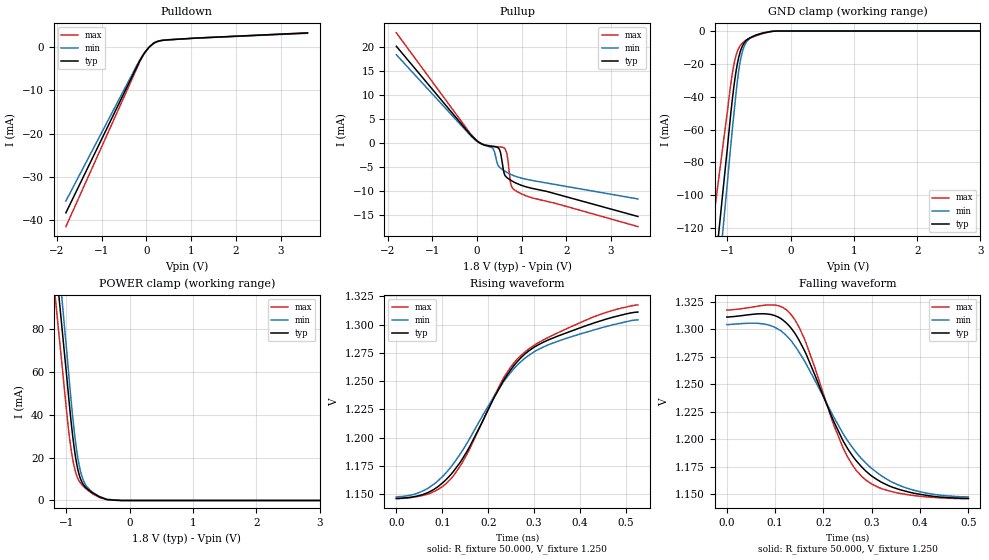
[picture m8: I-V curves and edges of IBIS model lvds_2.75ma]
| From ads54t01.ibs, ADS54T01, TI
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[Model]   lvds_2.75ma
Model_type 3-state
Vref=1.250E+00
Rref=5.000E+01
Cref=0.000E+00
Vmeas=1.250E+00
C_comp   7.860E-13   7.790E-13   7.930E-13
[Voltage Range]   1.800E+00   1.650E+00   1.950E+00
[POWER Clamp Reference]   1.800E+00   1.650E+00   1.950E+00
[GND Clamp Reference]   0.000E+00   0.000E+00   0.000E+00
[Pullup Reference]   1.800E+00   1.650E+00   1.950E+00
[Pulldown Reference]   0.000E+00   0.000E+00   0.000E+00
[Temperature Range]   25   85   -40
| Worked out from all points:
|   slope of the pulldown table from 0 to 0.27 V, typ, clamps not added: 125 ohm
|   slope of the pullup table from 0 to 0.27 V, typ, clamps not added: 263 ohm
|   GND clamp passes 1 mA (typ) near -0.41 V on its own axis
|   POWER clamp passes 1 mA (typ) near -0.41 V on its own axis
|   rising waveform, R_fixture 50.000, V_fixture 1.250: 20-80 % time 153ps typ, 161ps min, 159ps max; typ from 1.15 V to 1.31 V
|   falling waveform, R_fixture 50.000, V_fixture 1.250: 20-80 % time 107ps typ, 128ps min, 87.4ps max; typ from 1.31 V to 1.15 V
[GND Clamp]
-1.8V     -374.4mA   -423.5mA   -288.4mA
-1.02V    -78.69mA   -100.5mA   -54.92mA
-920mV    -41.17mA   -59.34mA   -25.51mA
-860mV    -23.88mA   -36.88mA   -14.48mA
-820mV    -15.94mA   -23.97mA   -10.43mA
-780mV    -10.76mA   -15.27mA   -8.038mA
-740mV    -7.589mA   -9.923mA   -6.562mA
-700mV    -5.657mA   -6.755mA   -5.499mA
-640mV    -4.069mA   -4.329mA   -4.359mA
-460mV    -1.489mA   -1.354mA   -1.806mA
-220mV    -4.201uA   -14.01uA   -11.29uA
3.6V      0A         0A         0A
[Power Clamp]
-1.8V     302.8mA    334.3mA    279.3mA
-1.76V    290.6mA    320.1mA    266.6mA
-1.06V    77.25mA    90.47mA    60.21mA
-940mV    40.5mA     50.88mA    26.54mA
-880mV    24.97mA    33.1mA     16.1mA
-820mV    14.43mA    19.78mA    10.24mA
-780mV    10.23mA    13.83mA    8.195mA
-720mV    6.913mA    8.542mA    6.262mA
-580mV    3.451mA    3.702mA    2.982mA
-360mV    441.4uA    538.8uA    356.5uA
-140mV    0A         9.789uA    18.55uA
3.6V      0A         0A         0A
[Pullup]
-1.81V    20.08mA    18.32mA    22.89mA
-30mV     557uA      470uA      670.5uA
350mV     -808.1uA   -1.098mA   -746.4uA
490mV     -1.233mA   -4.983mA   -882.3uA
530mV     -2.18mA    -5.333mA   -921.9uA
590mV     -5.61mA    -5.733mA   -1.023mA
630mV     -6.9mA     -5.977mA   -1.283mA
690mV     -7.445mA   -6.309mA   -3.393mA
750mV     -7.81mA    -6.595mA   -8.25mA
810mV     -8.14mA    -6.84mA    -9.667mA
1.23V     -9.53mA    -7.887mA   -11.51mA
3.61V     -15.41mA   -11.75mA   -17.51mA
[Pulldown]
-1.8V     -38.31mA   -35.57mA   -41.49mA
-140mV    -3.033mA   -2.834mA   -3.273mA
-40mV     -1.332mA   -1.268mA   -1.406mA
60mV      -43.2uA    -75.24uA   12.04uA
160mV     850.8uA    778.4uA    937.1uA
300mV     1.43mA     1.396mA    1.441mA
520mV     1.683mA    1.687mA    1.653mA
3.6V      3.242mA    3.167mA    3.272mA
[Rising Waveform]
R_fixture = 50.000
V_fixture = 1.250
V_fixture_min = 1.250
V_fixture_max = 1.250
|  time   V(typ)   V(min)   V(max)
0s        1.146V     1.147V     1.146V
68ps      1.151V     1.155V     1.15V
120ps     1.168V     1.175V     1.164V
156ps     1.189V     1.197V     1.187V
232ps     1.25V      1.248V     1.252V
256ps     1.264V     1.261V     1.266V
286ps     1.276V     1.272V     1.278V
336ps     1.287V     1.283V     1.29V
428ps     1.301V     1.295V     1.307V
526ps     1.311V     1.304V     1.317V
[Falling Waveform]
R_fixture = 50.000
V_fixture = 1.250
V_fixture_min = 1.250
V_fixture_max = 1.250
|  time   V(typ)   V(min)   V(max)
0s        1.311V     1.304V     1.317V
90ps      1.313V     1.303V     1.322V
112ps     1.31V      1.298V     1.321V
134ps     1.3V       1.289V     1.313V
164ps     1.278V     1.269V     1.288V
240ps     1.199V     1.206V     1.193V
264ps     1.183V     1.19V      1.174V
288ps     1.171V     1.178V     1.163V
372ps     1.153V     1.156V     1.15V
500ps     1.146V     1.147V     1.146V
[Ramp]
dV/dt_r   9.8940E-02/1.5250E-10   9.4020E-02/1.6090E-10   1.0290E-01/1.5850E-10
dV/dt_f   9.8940E-02/1.0691E-10   9.4020E-02/1.2806E-10   1.0290E-01/8.7078E-11
R_load = 50
